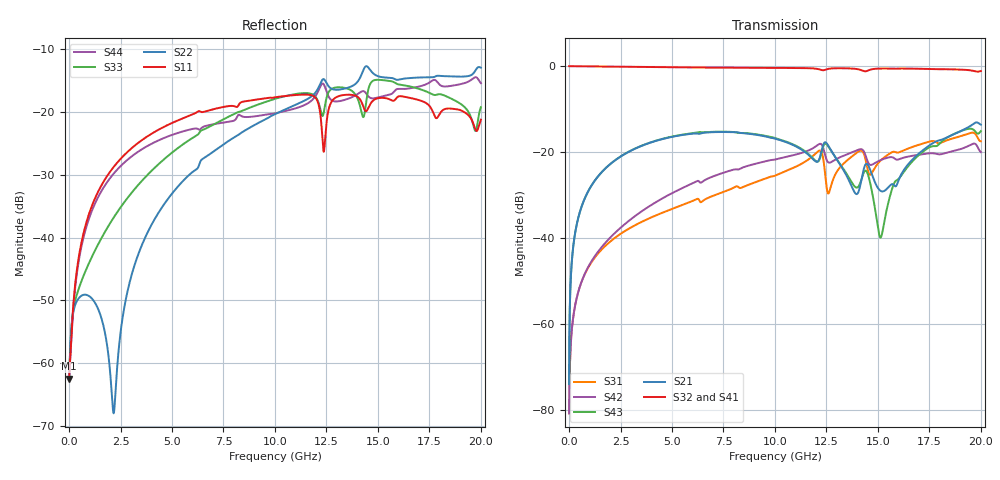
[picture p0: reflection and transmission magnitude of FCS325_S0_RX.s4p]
!Generated from:
! 1
! 2
! 3
! 4
!PowerSI Version: 17.0.2.03131.86335  002
!Computer Host Name: W764D-PINDIS
!TouchstoneFormatFlag = 1
! GNDNET
! NETSLIST
!User Comments:
!  Touchstone generated by fitter/viewer
#	Hz	S	RI	R	50
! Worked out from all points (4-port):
!   4999 points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, 4.001 MHz to 20 GHz, reference 50 ohm
!   strongest paths, dB at 4.001 MHz, 5.001 GHz, 10 GHz, 15 GHz, 20 GHz:
!     S32: 0.0, -0.3, -0.4, -0.6, -1.1
!     S41: 0.0, -0.3, -0.4, -0.5, -1.0
!     S21: -73.9, -16.4, -16.9, -28.3, -13.6
!     S43: -73.9, -16.4, -16.7, -37.6, -15.1
!     S42: -80.7, -29.5, -21.7, -22.1, -20.0
!     S31: -80.7, -33.2, -25.5, -22.6, -17.5
!   lowest |S11| = -62.5 dB at 4.001 MHz (marker M1), VSWR 1.00, Z = 50.1 + j0.00485 ohm
!   |S11| at or under -10 dB: start of sweep to end of sweep
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4000800  0.00075 4.85e-05  8.02e-05 0.000186  -7.85e-05 -4.86e-05  0.9992 -0.000982
         8.02e-05 0.000186  0.000753 0.00011  0.9992 -0.00092  -7.84e-05 -4.86e-05
         -7.85e-05 -4.86e-05  0.9992 -0.00092  0.000753 0.00011  8.02e-05 0.000186
         0.9992 -0.000982  -7.84e-05 -4.86e-05  8.02e-05 0.000186  0.00075 4.87e-05
5.681136e8  0.00312 -0.00796  0.00321 0.0215  -0.000865 -0.0028  0.9879 -0.1215
            0.00321 0.0215  0.00322 0.00111  0.989 -0.1132  -0.000656 -0.00286
            -0.000865 -0.0028  0.989 -0.1132  0.00422 0.00101  0.00323 0.0215
            0.9879 -0.1215  -0.000656 -0.00286  0.00323 0.0215  0.00211 -0.00768
2.164433e9  -0.00232 -0.0364  0.0343 0.0701  -0.00498 -0.00848  0.8855 -0.4346
            0.0343 0.0701  -6.14e-05 -0.000393  0.8997 -0.4067  -0.00306 -0.0107
            -0.00498 -0.00848  0.8997 -0.4067  0.0129 -0.0064  0.0348 0.0701
            0.8855 -0.4346  -0.00306 -0.0107  0.0348 0.0701  -0.0139 -0.0292
2.980596e9  -0.00975 -0.0496  0.0595 0.0845  -0.00815 -0.0104  0.7958 -0.574
            0.0595 0.0845  -0.00441 0.00146  0.8212 -0.54  -0.00603 -0.0153
            -0.00815 -0.0104  0.8212 -0.54  0.0176 -0.0134  0.0604 0.0844
            0.7958 -0.574  -0.00603 -0.0153  0.0604 0.0844  -0.0283 -0.0331
1.24825e10  -0.0554 -0.0519  0.1196 -0.0485  0.00814 0.0434  -0.7239 -0.5397
            0.1196 -0.0485  0.1369 0.1059  -0.6476 -0.6458  -0.00341 0.0846
            0.00814 0.0434  -0.6476 -0.6458  -0.0589 -0.1108  0.1055 -0.0665
            -0.7239 -0.5397  -0.00341 0.0846  0.1055 -0.0665  0.1248 0.082
1.513103e10  -0.1282 -0.0212  0.0351 0.00523  -0.0243 0.0762  -0.9459 -0.058
             0.0351 0.00523  0.1874 0.0358  -0.9035 -0.2529  0.00702 0.0807
             -0.0243 0.0762  -0.9035 -0.2529  -0.167 -0.0689  -0.0101 -0.000864
             -0.9459 -0.058  0.00702 0.0807  -0.0101 -0.000864  0.132 -0.0107
2e10  -0.0871 0.000593  0.1882 0.0902  0.1235 0.0513  -0.527 0.7184
      0.1882 0.0902  0.2214 -0.0458  -0.678 0.5567  0.0885 0.0468
      0.1235 0.0513  -0.678 0.5567  -0.0443 0.1003  0.125 0.1235
      -0.527 0.7184  0.0885 0.0468  0.125 0.1235  0.0336 -0.1668
